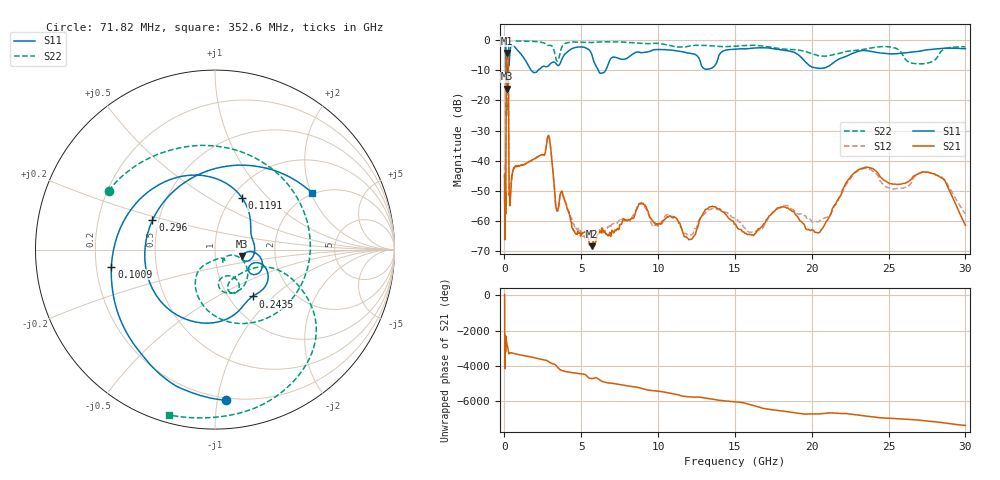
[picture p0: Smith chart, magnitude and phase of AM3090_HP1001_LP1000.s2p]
! Date/Time: Thu, Feb 28, 2019 2:03 PM
! Network Analyzer: Agilent Technologies E8364B Rev: A.07.50.67
! Sweep from 0.010 to 30.000 GHz, 1601 Points, Sweep Type: LOG
! Power Supply: 5.023 V, 0.002 A
# Hz S DB R 50
!freq MagS11 AngS11 MagS21 AngS21 MagS12 AngS12 MagS22 AngS22
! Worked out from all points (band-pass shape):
!   1601 points, 10 MHz to 30 GHz, reference 50 ohm
!   highest |S21| = -4.25 dB at 163.2 MHz (marker M1); lowest = -68.3 dB at 5.668 GHz (marker M2)
!   |S21| within 3 dB of the highest: 124.2 MHz to 242.7 MHz (118.5 MHz wide, 64.6 % of centre)
!   lowest |S11| = -16.1 dB at 154.4 MHz (marker M3), VSWR 1.37, Z = 67.7 - j5.06 ohm
!   |S11| at or under -10 dB: 119.5 MHz to 223.2 MHz (103.7 MHz wide, 60.5 % of centre); 1.743 GHz to 2.193 GHz (449.4 MHz wide, 22.8 % of centre); 6.102 GHz to 6.59 GHz (488 MHz wide, 7.69 % of centre)
!   |S22| runs from -25.5 to -0.1 dB; largest |S21 - S12| = 0.013
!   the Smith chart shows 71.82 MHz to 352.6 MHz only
!   S11 on the Smith chart (normalised r, x): 71.82 MHz: 0.18, -1.06; 100.9 MHz: 0.26, -0.08; 119.1 MHz: 1.11, +0.72; 243.5 MHz: 1.28, -0.75; 296 MHz: 0.46, +0.18; 352.6 MHz: 1.94, +2.03
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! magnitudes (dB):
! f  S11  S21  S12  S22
! 10 MHz  -0.3  -45.5  -41.3  -0.7
! 38.04 MHz  -0.5  -60.8  -58.6  -1.4
! 71.82 MHz  -1.5  -51.8  -51.2  -3.4
! 87.3 MHz  -2.8  -52.8  -54.8  -4.9
! 100.9 MHz  -4.7  -34.8  -34.6  -5.5
! 119.1 MHz  -9.8  -10.2  -10.2  -13.1
! 144.7 MHz  -14.4  -4.6  -4.6  -23.0
! 154.4 MHz  -16.1  -4.3  -4.3  -20.4
! 163.2 MHz  -14.4  -4.2  -4.2  -15.3
! 243.5 MHz  -9.5  -7.4  -7.3  -14.3
! 296 MHz  -8.3  -48.4  -48.4  -1.1
! 352.6 MHz  -4.1  -54.5  -53.4  -0.4
! 550.5 MHz  -1.9  -43.2  -43.3  -0.2
! 2.084 GHz  -10.6  -38.9  -38.9  -0.5
! 2.884 GHz  -8.4  -31.8  -31.7  -1.8
! 3.419 GHz  -8.2  -56.4  -56.7  -7.0
! 5.668 GHz  -4.5  -68.3  -64.7  -0.8
! 7.926 GHz  -6.2  -59.6  -59.6  -0.7
! 20.2 GHz  -9.2  -63.7  -60.0  -4.8
! 23.48 GHz  -3.5  -42.2  -42.5  -3.0
! 27.83 GHz  -3.1  -44.2  -44.0  -7.2
! 30 GHz  -2.9  -61.4  -57.6  -2.2
